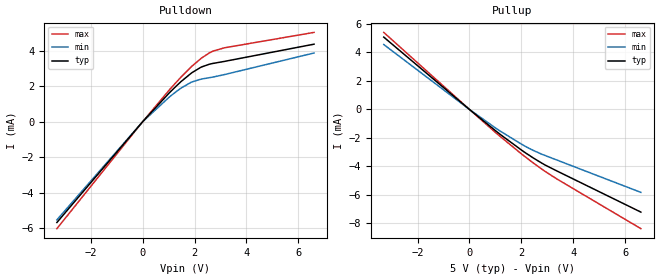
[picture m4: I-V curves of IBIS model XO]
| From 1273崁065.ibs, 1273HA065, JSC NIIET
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[Model]   XO
Model_type Output
Polarity   Non-Inverting
Vmeas =   1.65V
C_comp   7.970E-13F   7.970E-13F   7.970E-13F
[Temperature Range]   25   -60   85
[Voltage Range]   5.00V   4.50V   5.50V
[Pullup Reference]   5.00V   4.50V   5.50V
[Pulldown Reference]   0.00V   0.00V   0.00V
[POWER Clamp Reference]   5.00V   4.50V   5.50V
[GND Clamp Reference]   0.00V   0.00V   0.00V
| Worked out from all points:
|   slope of the pulldown table from 0 to 0.75 V, typ, clamps not added: 631 ohm
|   slope of the pullup table from 0 to 0.75 V, typ, clamps not added: 672 ohm
[Pullup]
| Voltage   I(typ)   I(min)   I(max)
-3.3V     5.079mA    4.558mA    5.41mA
0V        0A         0A         0A
980mV     -1.458mA   -1.272mA   -1.581mA
2.02V     -2.874mA   -2.455mA   -3.148mA
2.78V     -3.762mA   -3.14mA    -4.181mA
3.36V     -4.313mA   -3.546mA   -4.873mA
6.6V      -7.206mA   -5.821mA   -8.368mA
[Pulldown]
| Voltage   I(typ)   I(min)   I(max)
-3.3V     -5.677mA   -5.528mA   -6.025mA
0V        0A         0A         0A
1.04V     1.648mA    1.409mA    1.814mA
1.3V      2.019mA    1.709mA    2.235mA
1.86V     2.725mA    2.22mA     3.078mA
2.26V     3.087mA    2.407mA    3.584mA
2.7V      3.287mA    2.518mA    3.978mA
3.14V     3.401mA    2.657mA    4.168mA
6.6V      4.375mA    3.878mA    5.039mA
[Ramp]
| variable   typ   min   max
dV/dt_r   1.2201E-01/6.8672E-10   9.5023E-02/7.0313E-10   1.4565E-01/6.7039E-10
dV/dt_f   9.9371E-02/1.1356E-09   7.4630E-02/1.3731E-09   2.7600E+00/1.0589E-09
R_load = 50ohms
